DATA_BLOCK "Er"
TITLE =
VERSION : 0.1


  STRUCT
   KmA_DlmVF_GF { S7_m_c := 'true' }: BOOL ;	//GENERAL FAULT
   KmA_DlmVF_Strt { S7_m_c := 'true' }: BOOL ;	//FAULT START DELAY
   KmA_DlmVF_Stop { S7_m_c := 'true' }: BOOL ;	//FAULT STOP DELAY
   KmA_DlmVF_Trip { S7_m_c := 'true' }: BOOL ;	//FAULT TRIPPED
   KmA_Akt_GF { S7_m_c := 'true' }: BOOL ;	//GENERAL FAULT
   KmA_Akt_Strt { S7_m_c := 'true' }: BOOL ;	//FAULT START DELAY
   KmA_Akt_Stop { S7_m_c := 'true' }: BOOL ;	//FAULT STOP DELAY
   KmA_Akt_Trip { S7_m_c := 'true' }: BOOL ;	//FAULT TRIPPED
   KmA_SL_HL { S7_m_c := 'true' }: BOOL ;	//SILO HIGH LEVEL
   KmA_SL_LL { S7_m_c := 'true' }: BOOL ;	//SILO LOW LEVEL
   KmA_DlmKpk_GF { S7_m_c := 'true' }: BOOL ;	//GENERAL FAULT
   KmA_DlmKpk_Opn { S7_m_c := 'true' }: BOOL ;	//FAULT OPEN DELAY
   KmA_DlmKpk_Cls { S7_m_c := 'true' }: BOOL ;	//FAULT CLOSE DELAY
   KmA_DlmKpk_BthLmt { S7_m_c := 'true' }: BOOL ;	//BOTH LIMITS MADE
   KmA_BsltVF_GF { S7_m_c := 'true' }: BOOL ;	//GENERAL FAULT
   KmA_BsltVF_Strt { S7_m_c := 'true' }: BOOL ;	//FAULT START DELAY
   KmA_BsltVF_Stop { S7_m_c := 'true' }: BOOL ;	//FAULT STOP DELAY
   KmA_BsltVF_Trip { S7_m_c := 'true' }: BOOL ;	//FAULT TRIPPED
   KmA_BsltKpk_GF { S7_m_c := 'true' }: BOOL ;	//GENERAL FAULT
   KmA_BsltKpk_Opn { S7_m_c := 'true' }: BOOL ;	//FAULT OPEN DELAY
   KmA_BsltKpk_Cls { S7_m_c := 'true' }: BOOL ;	//FAULT CLOSE DELAY
   KmA_BsltKpk_BthLmt { S7_m_c := 'true' }: BOOL ;	//BOTH LIMITS MADE
   KmA_Ydk { S7_m_c := 'true' }: BOOL ;
   KmA_Ydk1 { S7_m_c := 'true' }: BOOL ;
   KmB_DlmVF_GF { S7_m_c := 'true' }: BOOL ;	//GENERAL FAULT
   KmB_DlmVF_Strt { S7_m_c := 'true' }: BOOL ;	//FAULT START DELAY
   KmB_DlmVF_Stop { S7_m_c := 'true' }: BOOL ;	//FAULT STOP DELAY
   KmB_DlmVF_Trip { S7_m_c := 'true' }: BOOL ;	//FAULT TRIPPED
   KmB_Akt_GF { S7_m_c := 'true' }: BOOL ;	//GENERAL FAULT
   KmB_Akt_Strt { S7_m_c := 'true' }: BOOL ;	//FAULT START DELAY
   KmB_Akt_Stop { S7_m_c := 'true' }: BOOL ;	//FAULT STOP DELAY
   KmB_Akt_Trip { S7_m_c := 'true' }: BOOL ;	//FAULT TRIPPED
   KmB_DlmKpk_GF { S7_m_c := 'true' }: BOOL ;	//GENERAL FAULT
   KmB_DlmKpk_Opn { S7_m_c := 'true' }: BOOL ;	//FAULT OPEN DELAY
   KmB_DlmKpk_Cls { S7_m_c := 'true' }: BOOL ;	//FAULT CLOSE DELAY
   KmB_DlmKpk_BthLmt { S7_m_c := 'true' }: BOOL ;	//BOTH LIMITS MADE
   KmB_SL_HL { S7_m_c := 'true' }: BOOL ;	//SILO HIGH LEVEL
   KmB_SL_LL { S7_m_c := 'true' }: BOOL ;	//SILO LOW LEVEL
   KmB_BsltVF_GF { S7_m_c := 'true' }: BOOL ;	//GENERAL FAULT
   KmB_BsltVF_Strt { S7_m_c := 'true' }: BOOL ;	//FAULT START DELAY
   KmB_BsltVF_Stop { S7_m_c := 'true' }: BOOL ;	//FAULT STOP DELAY
   KmB_BsltVF_Trip { S7_m_c := 'true' }: BOOL ;	//FAULT TRIPPED
   KmB_BsltKpk_GF { S7_m_c := 'true' }: BOOL ;	//GENERAL FAULT
   KmB_BsltKpk_Opn { S7_m_c := 'true' }: BOOL ;	//FAULT OPEN DELAY
   KmB_BsltKpk_Cls { S7_m_c := 'true' }: BOOL ;	//FAULT CLOSE DELAY
   KmB_BsltKpk_BthLmt { S7_m_c := 'true' }: BOOL ;	//BOTH LIMITS MADE
   KmB_Ydk { S7_m_c := 'true' }: BOOL ;
   KmB_Ydk1 { S7_m_c := 'true' }: BOOL ;
   SdA_DlmHlz_GF { S7_m_c := 'true' }: BOOL ;	//GENERAL FAULT
   SdA_DlmHlz_Strt { S7_m_c := 'true' }: BOOL ;	//FAULT START DELAY
   SdA_DlmHlz_Stop { S7_m_c := 'true' }: BOOL ;	//FAULT STOP DELAY
   SdA_DlmHlz_Trip { S7_m_c := 'true' }: BOOL ;	//FAULT TRIPPED
   SdA_Akt_GF { S7_m_c := 'true' }: BOOL ;	//GENERAL FAULT
   SdA_Akt_Strt { S7_m_c := 'true' }: BOOL ;	//FAULT START DELAY
   SdA_Akt_Stop { S7_m_c := 'true' }: BOOL ;	//FAULT STOP DELAY
   SdA_Akt_Trip { S7_m_c := 'true' }: BOOL ;	//FAULT TRIPPED
   SdA_SL_HL { S7_m_c := 'true' }: BOOL ;	//SILO HIGH LEVEL
   SdA_SL_LL { S7_m_c := 'true' }: BOOL ;	//SILO LOW LEVEL
   SdA_DlmKpk_GF { S7_m_c := 'true' }: BOOL ;	//GENERAL FAULT
   SdA_DlmKpk_Opn { S7_m_c := 'true' }: BOOL ;	//FAULT OPEN DELAY
   SdA_DlmKpk_Cls { S7_m_c := 'true' }: BOOL ;	//FAULT CLOSE DELAY
   SdA_DlmKpk_BthLmt { S7_m_c := 'true' }: BOOL ;	//BOTH LIMITS MADE
   SdB_DlmHlz_GF1 { S7_m_c := 'true' }: BOOL ;	//GENERAL FAULT
   SdB_DlmHlz_Strt { S7_m_c := 'true' }: BOOL ;	//FAULT START DELAY
   SdB_DlmHlz_Stop { S7_m_c := 'true' }: BOOL ;	//FAULT STOP DELAY
   SdB_DlmHlz_Trip { S7_m_c := 'true' }: BOOL ;	//FAULT TRIPPED
   SdB_Akt_GF { S7_m_c := 'true' }: BOOL ;	//GENERAL FAULT
   SdB_Akt_Strt { S7_m_c := 'true' }: BOOL ;	//FAULT START DELAY
   SdB_Akt_Stop { S7_m_c := 'true' }: BOOL ;	//FAULT STOP DELAY
   SdB_Akt_Trip { S7_m_c := 'true' }: BOOL ;	//FAULT TRIPPED
   SdB_SL_HL { S7_m_c := 'true' }: BOOL ;	//SILO HIGH LEVEL
   SdB_SL_LL { S7_m_c := 'true' }: BOOL ;	//SILO LOW LEVEL
   SdB_DlmKpk_GF { S7_m_c := 'true' }: BOOL ;	//GENERAL FAULT
   SdB_DlmKpk_Opn { S7_m_c := 'true' }: BOOL ;	//FAULT OPEN DELAY
   SdB_DlmKpk_Cls { S7_m_c := 'true' }: BOOL ;	//FAULT CLOSE DELAY
   SdB_DlmKpk_BthLmt { S7_m_c := 'true' }: BOOL ;	//BOTH LIMITS MADE
   Sd_BsltVF_GF { S7_m_c := 'true' }: BOOL ;	//GENERAL FAULT
   Sd_BsltVF_Strt { S7_m_c := 'true' }: BOOL ;	//FAULT START DELAY
   Sd_BsltVF_Stop { S7_m_c := 'true' }: BOOL ;	//FAULT STOP DELAY
   Sd_BsltVF_Trip { S7_m_c := 'true' }: BOOL ;	//FAULT TRIPPED
   Sd_BsltKpk_GF { S7_m_c := 'true' }: BOOL ;	//GENERAL FAULT
   Sd_BsltKpk_Opn { S7_m_c := 'true' }: BOOL ;	//FAULT OPEN DELAY
   Sd_BsltKpk_Cls { S7_m_c := 'true' }: BOOL ;	//FAULT CLOSE DELAY
   Sd_BsltKpk_BthLmt { S7_m_c := 'true' }: BOOL ;	//BOTH LIMITS MADE
   Sd_Ydk { S7_m_c := 'true' }: BOOL ;
   Sd_Ydk1 { S7_m_c := 'true' }: BOOL ;
   Sd_Ydk2 { S7_m_c := 'true' }: BOOL ;
   Sd_Ydk3 { S7_m_c := 'true' }: BOOL ;
   DlA_DlmHlz_GF { S7_m_c := 'true' }: BOOL ;	//GENERAL FAULT
   DlA_DlmHlz_Strt { S7_m_c := 'true' }: BOOL ;	//FAULT START DELAY
   DlA_DlmHlz_Stop { S7_m_c := 'true' }: BOOL ;	//FAULT STOP DELAY
   DlA_DlmHlz_Trip { S7_m_c := 'true' }: BOOL ;	//FAULT TRIPPED
   DlA_Akt_GF { S7_m_c := 'true' }: BOOL ;	//GENERAL FAULT
   DlA_Akt_Strt { S7_m_c := 'true' }: BOOL ;	//FAULT START DELAY
   DlA_Akt_Stop { S7_m_c := 'true' }: BOOL ;	//FAULT STOP DELAY
   DlA_Akt_Trip { S7_m_c := 'true' }: BOOL ;	//FAULT TRIPPED
   DlA_SL_HL { S7_m_c := 'true' }: BOOL ;	//SILO HIGH LEVEL
   DlA_SL_LL { S7_m_c := 'true' }: BOOL ;	//SILO LOW LEVEL
   DlA_DlmKpk_GF { S7_m_c := 'true' }: BOOL ;	//GENERAL FAULT
   DlA_DlmKpk_Opn { S7_m_c := 'true' }: BOOL ;	//FAULT OPEN DELAY
   DlA_DlmKpk_Cls { S7_m_c := 'true' }: BOOL ;	//FAULT CLOSE DELAY
   DlA_DlmKpk_BthLmt { S7_m_c := 'true' }: BOOL ;	//BOTH LIMITS MADE
   DlB_DlmHlz_GF { S7_m_c := 'true' }: BOOL ;	//GENERAL FAULT
   DlB_DlmHlz_Strt { S7_m_c := 'true' }: BOOL ;	//FAULT START DELAY
   DlB_DlmHlz_Stop { S7_m_c := 'true' }: BOOL ;	//FAULT STOP DELAY
   DlB_DlmHlz_Trip { S7_m_c := 'true' }: BOOL ;	//FAULT TRIPPED
   DlB_Akt_GF { S7_m_c := 'true' }: BOOL ;	//GENERAL FAULT
   DlB_Akt_Strt { S7_m_c := 'true' }: BOOL ;	//FAULT START DELAY
   DlB_Akt_Stop { S7_m_c := 'true' }: BOOL ;	//FAULT STOP DELAY
   DlB_Akt_Trip { S7_m_c := 'true' }: BOOL ;	//FAULT TRIPPED
   DlB_SL_HL { S7_m_c := 'true' }: BOOL ;	//SILO HIGH LEVEL
   DlB_SL_LL { S7_m_c := 'true' }: BOOL ;	//SILO LOW LEVEL
   DlB_DlmKpk_GF { S7_m_c := 'true' }: BOOL ;	//GENERAL FAULT
   DlB_DlmKpk_Opn { S7_m_c := 'true' }: BOOL ;	//FAULT OPEN DELAY
   DlB_DlmKpk_Cls { S7_m_c := 'true' }: BOOL ;	//FAULT CLOSE DELAY
   DlB_DlmKpk_BthLmt { S7_m_c := 'true' }: BOOL ;	//BOTH LIMITS MADE
   Dl_BsltHlz1_GF { S7_m_c := 'true' }: BOOL ;	//GENERAL FAULT
   Dl_BsltHlz1_Strt { S7_m_c := 'true' }: BOOL ;	//FAULT START DELAY
   Dl_BsltHlz1_Stop { S7_m_c := 'true' }: BOOL ;	//FAULT STOP DELAY
   Dl_BsltHlz1_Trip { S7_m_c := 'true' }: BOOL ;	//FAULT TRIPPED
   Dl_BsltHlz2_GF { S7_m_c := 'true' }: BOOL ;	//GENERAL FAULT
   Dl_BsltHlz2_Strt { S7_m_c := 'true' }: BOOL ;	//FAULT START DELAY
   Dl_BsltHlz2_Stop { S7_m_c := 'true' }: BOOL ;	//FAULT STOP DELAY
   Dl_BsltHlz2_Trip { S7_m_c := 'true' }: BOOL ;	//FAULT TRIPPED
   Dl_BsltKpk_GF { S7_m_c := 'true' }: BOOL ;	//GENERAL FAULT
   Dl_BsltKpk_Opn { S7_m_c := 'true' }: BOOL ;	//FAULT OPEN DELAY
   Dl_BsltKpk_Cls { S7_m_c := 'true' }: BOOL ;	//FAULT CLOSE DELAY
   Dl_BsltKpk_BthLmt { S7_m_c := 'true' }: BOOL ;	//BOTH LIMITS MADE
   Kl_DlmHlz_GF { S7_m_c := 'true' }: BOOL ;	//GENERAL FAULT
   Kl_DlmHlz_Strt { S7_m_c := 'true' }: BOOL ;	//FAULT START DELAY
   Kl_DlmHlz_Stop { S7_m_c := 'true' }: BOOL ;	//FAULT STOP DELAY
   Kl_DlmHlz_Trip { S7_m_c := 'true' }: BOOL ;	//FAULT TRIPPED
   Kl_Akt_GF { S7_m_c := 'true' }: BOOL ;	//GENERAL FAULT
   Kl_Akt_Strt { S7_m_c := 'true' }: BOOL ;	//FAULT START DELAY
   Kl_Akt_Stop { S7_m_c := 'true' }: BOOL ;	//FAULT STOP DELAY
   Kl_Akt_Trip { S7_m_c := 'true' }: BOOL ;	//FAULT TRIPPED
   Kl_SL_HL { S7_m_c := 'true' }: BOOL ;	//SILO HIGH LEVEL
   Kl_SL_LL { S7_m_c := 'true' }: BOOL ;	//SILO LOW LEVEL
   Kl_DlmKpk_GF { S7_m_c := 'true' }: BOOL ;	//GENERAL FAULT
   Kl_DlmKpk_Opn { S7_m_c := 'true' }: BOOL ;	//FAULT OPEN DELAY
   Kl_DlmKpk_Cls { S7_m_c := 'true' }: BOOL ;	//FAULT CLOSE DELAY
   Kl_DlmKpk_BthLmt { S7_m_c := 'true' }: BOOL ;	//BOTH LIMITS MADE
   Kl_BsltVF_GF { S7_m_c := 'true' }: BOOL ;	//GENERAL FAULT
   Kl_BsltVF_Strt { S7_m_c := 'true' }: BOOL ;	//FAULT START DELAY
   Kl_BsltVF_Stop { S7_m_c := 'true' }: BOOL ;	//FAULT STOP DELAY
   Kl_BsltVF_Trip { S7_m_c := 'true' }: BOOL ;	//FAULT TRIPPED
   Kl_BsltKpk_GF { S7_m_c := 'true' }: BOOL ;	//GENERAL FAULT
   Kl_BsltKpk_Opn { S7_m_c := 'true' }: BOOL ;	//FAULT OPEN DELAY
   Kl_BsltKpk_Cls { S7_m_c := 'true' }: BOOL ;	//FAULT CLOSE DELAY
   Kl_BsltKpk_BthLmt { S7_m_c := 'true' }: BOOL ;	//BOTH LIMITS MADE
   Kl_Ydk { S7_m_c := 'true' }: BOOL ;
   Kl_Ydk1 { S7_m_c := 'true' }: BOOL ;
   FlA_DlmHlz_GF { S7_m_c := 'true' }: BOOL ;	//GENERAL FAULT
   FlA_DlmHlz_Strt { S7_m_c := 'true' }: BOOL ;	//FAULT START DELAY
   FlA_DlmHlz_Stop { S7_m_c := 'true' }: BOOL ;	//FAULT STOP DELAY
   FlA_DlmHlz_Trip { S7_m_c := 'true' }: BOOL ;	//FAULT TRIPPED
   FlA_Akt_GF { S7_m_c := 'true' }: BOOL ;	//GENERAL FAULT
   FlA_Akt_Strt { S7_m_c := 'true' }: BOOL ;	//FAULT START DELAY
   FlA_Akt_Stop { S7_m_c := 'true' }: BOOL ;	//FAULT STOP DELAY
   FlA_Akt_Trip { S7_m_c := 'true' }: BOOL ;	//FAULT TRIPPED
   FlA_SL_HL { S7_m_c := 'true' }: BOOL ;	//SILO HIGH LEVEL
   FlA_SL_LL { S7_m_c := 'true' }: BOOL ;	//SILO LOW LEVEL
   FlA_DlmKpk_GF { S7_m_c := 'true' }: BOOL ;	//GENERAL FAULT
   FlA_DlmKpk_Opn { S7_m_c := 'true' }: BOOL ;	//FAULT OPEN DELAY
   FlA_DlmKpk_Cls { S7_m_c := 'true' }: BOOL ;	//FAULT CLOSE DELAY
   FlA_DlmKpk_BthLmt { S7_m_c := 'true' }: BOOL ;	//BOTH LIMITS MADE
   FlB_DlmHlz_GF { S7_m_c := 'true' }: BOOL ;	//GENERAL FAULT
   FlB_DlmHlz_Strt { S7_m_c := 'true' }: BOOL ;	//FAULT START DELAY
   FlB_DlmHlz_Stop { S7_m_c := 'true' }: BOOL ;	//FAULT STOP DELAY
   FlB_DlmHlz_Trip { S7_m_c := 'true' }: BOOL ;	//FAULT TRIPPED
   FlB_Akt_GF { S7_m_c := 'true' }: BOOL ;	//GENERAL FAULT
   FlB_Akt_Strt { S7_m_c := 'true' }: BOOL ;	//FAULT START DELAY
   FlB_Akt_Stop { S7_m_c := 'true' }: BOOL ;	//FAULT STOP DELAY
   FlB_Akt_Trip { S7_m_c := 'true' }: BOOL ;	//FAULT TRIPPED
   FlB_SL_HL { S7_m_c := 'true' }: BOOL ;	//SILO HIGH LEVEL
   FlB_SL_LL { S7_m_c := 'true' }: BOOL ;	//SILO LOW LEVEL
   FlB_DlmKpk_GF { S7_m_c := 'true' }: BOOL ;	//GENERAL FAULT
   FlB_DlmKpk_Opn { S7_m_c := 'true' }: BOOL ;	//FAULT OPEN DELAY
   FlB_DlmKpk_Cls { S7_m_c := 'true' }: BOOL ;	//FAULT CLOSE DELAY
   FlB_DlmKpk_BthLmt { S7_m_c := 'true' }: BOOL ;	//BOTH LIMITS MADE
   Fl_BsltVF_GF { S7_m_c := 'true' }: BOOL ;	//GENERAL FAULT
   Fl_BsltVF_Strt { S7_m_c := 'true' }: BOOL ;	//FAULT START DELAY
   Fl_BsltVF_Stop { S7_m_c := 'true' }: BOOL ;	//FAULT STOP DELAY
   Fl_BsltVF_Trip { S7_m_c := 'true' }: BOOL ;	//FAULT TRIPPED
   Fl_BsltKpk_GF { S7_m_c := 'true' }: BOOL ;	//GENERAL FAULT
   Fl_BsltKpk_Opn { S7_m_c := 'true' }: BOOL ;	//FAULT OPEN DELAY
   Fl_BsltKpk_Cls { S7_m_c := 'true' }: BOOL ;	//FAULT CLOSE DELAY
   Fl_BsltKpk_BthLmt { S7_m_c := 'true' }: BOOL ;	//BOTH LIMITS MADE
   Fl_Ydk { S7_m_c := 'true' }: BOOL ;
   Fl_Ydk1 { S7_m_c := 'true' }: BOOL ;
   Fl_Ydk2 { S7_m_c := 'true' }: BOOL ;
   Fl_Ydk3 { S7_m_c := 'true' }: BOOL ;
   Sl_DlmHlz_GF { S7_m_c := 'true' }: BOOL ;	//GENERAL FAULT
   Sl_DlmHlz_Strt { S7_m_c := 'true' }: BOOL ;	//FAULT START DELAY
   Sl_DlmHlz_Stop { S7_m_c := 'true' }: BOOL ;	//FAULT STOP DELAY
   Sl_DlmHlz_Trip { S7_m_c := 'true' }: BOOL ;	//FAULT TRIPPED
   Sl_Akt_GF { S7_m_c := 'true' }: BOOL ;	//GENERAL FAULT
   Sl_Akt_Strt { S7_m_c := 'true' }: BOOL ;	//FAULT START DELAY
   Sl_Akt_Stop { S7_m_c := 'true' }: BOOL ;	//FAULT STOP DELAY
   Sl_Akt_Trip { S7_m_c := 'true' }: BOOL ;	//FAULT TRIPPED
   Sl_SL_HL { S7_m_c := 'true' }: BOOL ;	//SILO HIGH LEVEL
   Sl_SL_LL { S7_m_c := 'true' }: BOOL ;	//SILO LOW LEVEL
   Sl_DlmKpk_GF { S7_m_c := 'true' }: BOOL ;	//GENERAL FAULT
   Sl_DlmKpk_Opn { S7_m_c := 'true' }: BOOL ;	//FAULT OPEN DELAY
   Sl_DlmKpk_Cls { S7_m_c := 'true' }: BOOL ;	//FAULT CLOSE DELAY
   Sl_DlmKpk_BthLmt { S7_m_c := 'true' }: BOOL ;	//BOTH LIMITS MADE
   Sl_BsltVF_GF { S7_m_c := 'true' }: BOOL ;	//GENERAL FAULT
   Sl_BsltVF_Strt { S7_m_c := 'true' }: BOOL ;	//FAULT START DELAY
   Sl_BsltVF_Stop { S7_m_c := 'true' }: BOOL ;	//FAULT STOP DELAY
   Sl_BsltVF_Trip { S7_m_c := 'true' }: BOOL ;	//FAULT TRIPPED
   Sl_BsltKpk_GF { S7_m_c := 'true' }: BOOL ;	//GENERAL FAULT
   Sl_BsltKpk_Opn { S7_m_c := 'true' }: BOOL ;	//FAULT OPEN DELAY
   Sl_BsltKpk_Cls { S7_m_c := 'true' }: BOOL ;	//FAULT CLOSE DELAY
   Sl_BsltKpk_BthLmt { S7_m_c := 'true' }: BOOL ;	//BOTH LIMITS MADE
   Sl_Ydk { S7_m_c := 'true' }: BOOL ;
   Sl_Ydk1 { S7_m_c := 'true' }: BOOL ;
   Hm_DlmHlz_GF { S7_m_c := 'true' }: BOOL ;	//GENERAL FAULT
   Hm_DlmHlz_Strt { S7_m_c := 'true' }: BOOL ;	//FAULT START DELAY
   Hm_DlmHlz_Stop { S7_m_c := 'true' }: BOOL ;	//FAULT STOP DELAY
   Hm_DlmHlz_Trip { S7_m_c := 'true' }: BOOL ;	//FAULT TRIPPED
   Hm_Akt_GF { S7_m_c := 'true' }: BOOL ;	//GENERAL FAULT
   Hm_Akt_Strt { S7_m_c := 'true' }: BOOL ;	//FAULT START DELAY
   Hm_Akt_Stop { S7_m_c := 'true' }: BOOL ;	//FAULT STOP DELAY
   Hm_Akt_Trip { S7_m_c := 'true' }: BOOL ;	//FAULT TRIPPED
   Hm_SL_HL { S7_m_c := 'true' }: BOOL ;	//SILO HIGH LEVEL
   Hm_SL_LL { S7_m_c := 'true' }: BOOL ;	//SILO LOW LEVEL
   Hm_DlmKpk_GF { S7_m_c := 'true' }: BOOL ;	//GENERAL FAULT
   Hm_DlmKpk_Opn { S7_m_c := 'true' }: BOOL ;	//FAULT OPEN DELAY
   Hm_DlmKpk_Cls { S7_m_c := 'true' }: BOOL ;	//FAULT CLOSE DELAY
   Hm_DlmKpk_BthLmt { S7_m_c := 'true' }: BOOL ;	//BOTH LIMITS MADE
   Hm_BsltVF_GF { S7_m_c := 'true' }: BOOL ;	//GENERAL FAULT
   Hm_BsltVF_Strt { S7_m_c := 'true' }: BOOL ;	//FAULT START DELAY
   Hm_BsltVF_Stop { S7_m_c := 'true' }: BOOL ;	//FAULT STOP DELAY
   Hm_BsltVF_Trip { S7_m_c := 'true' }: BOOL ;	//FAULT TRIPPED
   Hm_BsltKpk_GF { S7_m_c := 'true' }: BOOL ;	//GENERAL FAULT
   Hm_BsltKpk_Opn { S7_m_c := 'true' }: BOOL ;	//FAULT OPEN DELAY
   Hm_BsltKpk_Cls { S7_m_c := 'true' }: BOOL ;	//FAULT CLOSE DELAY
   Hm_BsltKpk_BthLmt { S7_m_c := 'true' }: BOOL ;	//BOTH LIMITS MADE
   Hm_Ydk { S7_m_c := 'true' }: BOOL ;
   Hm_Ydk1 { S7_m_c := 'true' }: BOOL ;
   An_DlmHlz_GF { S7_m_c := 'true' }: BOOL ;	//GENERAL FAULT
   An_DlmHlz_Strt { S7_m_c := 'true' }: BOOL ;	//FAULT START DELAY
   An_DlmHlz_Stop { S7_m_c := 'true' }: BOOL ;	//FAULT STOP DELAY
   An_DlmHlz_Trip { S7_m_c := 'true' }: BOOL ;	//FAULT TRIPPED
   An_Akt_GF { S7_m_c := 'true' }: BOOL ;	//GENERAL FAULT
   An_Akt_Strt { S7_m_c := 'true' }: BOOL ;	//FAULT START DELAY
   An_Akt_Stop { S7_m_c := 'true' }: BOOL ;	//FAULT STOP DELAY
   An_Akt_Trip { S7_m_c := 'true' }: BOOL ;	//FAULT TRIPPED
   An_SL_HL { S7_m_c := 'true' }: BOOL ;	//SILO HIGH LEVEL
   An_SL_LL { S7_m_c := 'true' }: BOOL ;	//SILO LOW LEVEL
   An_DlmKpk_GF { S7_m_c := 'true' }: BOOL ;	//GENERAL FAULT
   An_DlmKpk_Opn { S7_m_c := 'true' }: BOOL ;	//FAULT OPEN DELAY
   An_DlmKpk_Cls { S7_m_c := 'true' }: BOOL ;	//FAULT CLOSE DELAY
   An_DlmKpk_BthLmt { S7_m_c := 'true' }: BOOL ;	//BOTH LIMITS MADE
   An_BsltKrs_GF { S7_m_c := 'true' }: BOOL ;	//GENERAL FAULT
   An_BsltKrs_Strt { S7_m_c := 'true' }: BOOL ;	//FAULT START DELAY
   An_BsltKrs_Stop { S7_m_c := 'true' }: BOOL ;	//FAULT STOP DELAY
   An_BsltKrs_Trip { S7_m_c := 'true' }: BOOL ;	//FAULT TRIPPED
   An_BsltHlz_GF { S7_m_c := 'true' }: BOOL ;	//GENERAL FAULT
   An_BsltHlz_Strt { S7_m_c := 'true' }: BOOL ;	//FAULT START DELAY
   An_BsltHlz_Stop { S7_m_c := 'true' }: BOOL ;	//FAULT STOP DELAY
   An_BsltHlz_Trip { S7_m_c := 'true' }: BOOL ;	//FAULT TRIPPED
   An_BsltKpk_GF { S7_m_c := 'true' }: BOOL ;	//GENERAL FAULT
   An_BsltKpk_Opn { S7_m_c := 'true' }: BOOL ;	//FAULT OPEN DELAY
   An_BsltKpk_Cls { S7_m_c := 'true' }: BOOL ;	//FAULT CLOSE DELAY
   An_BsltKpk_BthLmt { S7_m_c := 'true' }: BOOL ;	//BOTH LIMITS MADE
   An_Ydk { S7_m_c := 'true' }: BOOL ;
   An_Ydk1 { S7_m_c := 'true' }: BOOL ;
   An_Ydk2 { S7_m_c := 'true' }: BOOL ;
   An_Ydk3 { S7_m_c := 'true' }: BOOL ;
   An_Ydk4 { S7_m_c := 'true' }: BOOL ;
   An_Ydk5 { S7_m_c := 'true' }: BOOL ;
   e83_TopBnd_GF { S7_m_c := 'true' }: BOOL ;	//GENERAL FAULT
   e83_TopBnd_Strt { S7_m_c := 'true' }: BOOL ;	//FAULT START DELAY
   e83_TopBnd_Stop { S7_m_c := 'true' }: BOOL ;	//FAULT STOP DELAY
   e83_TopBnd_Trip { S7_m_c := 'true' }: BOOL ;	//FAULT TRIPPED
   e83_LmtSwtch { S7_m_c := 'true' }: BOOL ;	//CONVEYOR BAND LIMIT SWITCH ERROR
   e83_EmrSwtch { S7_m_c := 'true' }: BOOL ;	//CONVEYOR BAND EMERGENCY SWITCH ERROR
   e83_MovingSnsr { S7_m_c := 'true' }: BOOL ;	//CONVEYOR BAND MOVING SENSOR ERROR
   e83_Ydk { S7_m_c := 'true' }: BOOL ;	//CONVEYOR BAND MOVING SENSOR ERROR
   e83_Fan_GF { S7_m_c := 'true' }: BOOL ;	//GENERAL FAULT
   e83_Fan_Strt { S7_m_c := 'true' }: BOOL ;	//FAULT START DELAY
   e83_Fan_Stop { S7_m_c := 'true' }: BOOL ;	//FAULT STOP DELAY
   e83_Fan_Trip { S7_m_c := 'true' }: BOOL ;	//FAULT TRIPPED
   e83_Ydk1 { S7_m_c := 'true' }: BOOL ;	//CONVEYOR BAND MOVING SENSOR ERROR
   e83_Ydk2 { S7_m_c := 'true' }: BOOL ;	//CONVEYOR BAND MOVING SENSOR ERROR
   e83_Ydk3 { S7_m_c := 'true' }: BOOL ;	//CONVEYOR BAND MOVING SENSOR ERROR
   e83_Ydk4 { S7_m_c := 'true' }: BOOL ;	//CONVEYOR BAND MOVING SENSOR ERROR
   e87_Bnd_GF { S7_m_c := 'true' }: BOOL ;	//GENERAL FAULT
   e87_Bnd_Strt { S7_m_c := 'true' }: BOOL ;	//FAULT START DELAY
   e87_Bnd_Stop { S7_m_c := 'true' }: BOOL ;	//FAULT STOP DELAY
   e87_Bnd_Trip { S7_m_c := 'true' }: BOOL ;	//FAULT TRIPPED
   e87_LmtSwtch { S7_m_c := 'true' }: BOOL ;	//CONVEYOR BAND LIMIT SWITCH ERROR
   e87_EmrSwtch { S7_m_c := 'true' }: BOOL ;	//CONVEYOR BAND EMERGENCY SWITCH ERROR
   e87_MovingSnsr { S7_m_c := 'true' }: BOOL ;	//CONVEYOR BAND MOVING SENSOR ERROR
   e87_Ydk { S7_m_c := 'true' }: BOOL ;	//CONVEYOR BAND MOVING SENSOR ERROR
   e87_Fan_GF { S7_m_c := 'true' }: BOOL ;	//GENERAL FAULT
   e87_Fan_Strt { S7_m_c := 'true' }: BOOL ;	//FAULT START DELAY
   e87_Fan_Stop { S7_m_c := 'true' }: BOOL ;	//FAULT STOP DELAY
   e87_Fan_Trip { S7_m_c := 'true' }: BOOL ;	//FAULT TRIPPED
   e87_Ydk1 { S7_m_c := 'true' }: BOOL ;	//CONVEYOR BAND MOVING SENSOR ERROR
   e87_Ydk2 { S7_m_c := 'true' }: BOOL ;	//CONVEYOR BAND MOVING SENSOR ERROR
   e87_Ydk3 { S7_m_c := 'true' }: BOOL ;	//CONVEYOR BAND MOVING SENSOR ERROR
   e87_Ydk4 { S7_m_c := 'true' }: BOOL ;	//CONVEYOR BAND MOVING SENSOR ERROR
   TozTopFan_GF1 { S7_m_c := 'true' }: BOOL ;	//GENERAL FAULT
   TozTopFan_Strt1 { S7_m_c := 'true' }: BOOL ;	//FAULT START DELAY
   TozTopFan_Stop1 { S7_m_c := 'true' }: BOOL ;	//FAULT STOP DELAY
   TozTopFan_Trip1 { S7_m_c := 'true' }: BOOL ;	//FAULT TRIPPED
   Ydk { S7_m_c := 'true' }: BOOL ;	//FAULT TRIPPED
   Ydk1 { S7_m_c := 'true' }: BOOL ;	//FAULT TRIPPED
   Ydk2 { S7_m_c := 'true' }: BOOL ;	//FAULT TRIPPED
   Ydk3 { S7_m_c := 'true' }: BOOL ;	//FAULT TRIPPED
   TolErrKmADlm { S7_m_c := 'true' }: BOOL ;	//TOLERANS ERROR FILLING
   TolErrKmABslt { S7_m_c := 'true' }: BOOL ;	//TOLERANS ERROR DISCHARGE
   TolErrKmBDlm { S7_m_c := 'true' }: BOOL ;	//TOLERANS ERROR FILLING
   TolErrKmBBslt { S7_m_c := 'true' }: BOOL ;	//TOLERANS ERROR DISCHARGE
   TolErrSdADlm { S7_m_c := 'true' }: BOOL ;	//TOLERANS ERROR FILLING
   TolErrSdBDlm { S7_m_c := 'true' }: BOOL ;	//TOLERANS ERROR FILLING
   TolErrSdBslt { S7_m_c := 'true' }: BOOL ;	//TOLERANS ERROR DISCHARGE
   TolErrDlADlm { S7_m_c := 'true' }: BOOL ;	//TOLERANS ERROR FILLING
   TolErrDlBDlm { S7_m_c := 'true' }: BOOL ;	//TOLERANS ERROR FILLING
   TolErrDlBslt { S7_m_c := 'true' }: BOOL ;	//TOLERANS ERROR DISCHARGE
   TolErrKlDlm { S7_m_c := 'true' }: BOOL ;	//TOLERANS ERROR FILLING
   TolErrKlBslt { S7_m_c := 'true' }: BOOL ;	//TOLERANS ERROR DISCHARGE
   TolErrFlADlm { S7_m_c := 'true' }: BOOL ;	//TOLERANS ERROR FILLING
   TolErrFlBDlm { S7_m_c := 'true' }: BOOL ;	//TOLERANS ERROR FILLING
   TolErrFlBslt { S7_m_c := 'true' }: BOOL ;	//TOLERANS ERROR DISCHARGE
   TolErrSlDlm { S7_m_c := 'true' }: BOOL ;	//TOLERANS ERROR FILLING
   TolErrSlBslt { S7_m_c := 'true' }: BOOL ;	//TOLERANS ERROR DISCHARGE
   TolErrHmDlm { S7_m_c := 'true' }: BOOL ;	//TOLERANS ERROR FILLING
   TolErrHmBslt { S7_m_c := 'true' }: BOOL ;	//TOLERANS ERROR DISCHARGE
   TolErrAnDlm { S7_m_c := 'true' }: BOOL ;	//TOLERANS ERROR FILLING
   TolErrAnBslt { S7_m_c := 'true' }: BOOL ;	//TOLERANS ERROR DISCHARGE
   TolErrTopKntr { S7_m_c := 'true' }: BOOL ;	//TOLERANS ERROR
   TolErrYdk { S7_m_c := 'true' }: BOOL ;	//TOLERANS ERROR
   TolErrYdk1 { S7_m_c := 'true' }: BOOL ;	//TOLERANS ERROR
   BX3_ErrKmA { S7_m_c := 'true' }: BOOL ;	//BX3 ERROR
   BX3_ErrKmB { S7_m_c := 'true' }: BOOL ;	//BX3 ERROR
   BX3_ErrSd { S7_m_c := 'true' }: BOOL ;	//BX3 ERROR
   BX3_ErrDl { S7_m_c := 'true' }: BOOL ;	//BX3 ERROR
   BX3_ErrKl { S7_m_c := 'true' }: BOOL ;	//BX3 ERROR
   BX3_ErrFl { S7_m_c := 'true' }: BOOL ;	//BX3 ERROR
   BX3_ErrSl { S7_m_c := 'true' }: BOOL ;	//BX3 ERROR
   BX3_ErrHm { S7_m_c := 'true' }: BOOL ;	//BX3 ERROR
   BX3_ErrAn { S7_m_c := 'true' }: BOOL ;	//BX3 ERROR
   BX3_ErrYdk { S7_m_c := 'true' }: BOOL ;	//BX3 ERROR
   BX3_ErrYdk1 { S7_m_c := 'true' }: BOOL ;	//BX3 ERROR
   BX3_ErrYdk2 { S7_m_c := 'true' }: BOOL ;	//BX3 ERROR
   BX3_ErrYdk3 { S7_m_c := 'true' }: BOOL ;	//BX3 ERROR
   BX3_ErrYdk4 { S7_m_c := 'true' }: BOOL ;	//BX3 ERROR
   BX3_ErrYdk5 { S7_m_c := 'true' }: BOOL ;	//BX3 ERROR
   BX3_ErrYdk6 { S7_m_c := 'true' }: BOOL ;	//BX3 ERROR
  END_STRUCT ;
BEGIN
   KmA_DlmVF_GF := FALSE;
   KmA_DlmVF_Strt := FALSE;
   KmA_DlmVF_Stop := FALSE;
   KmA_DlmVF_Trip := FALSE;
   KmA_Akt_GF := FALSE;
   KmA_Akt_Strt := FALSE;
   KmA_Akt_Stop := FALSE;
   KmA_Akt_Trip := FALSE;
   KmA_SL_HL := FALSE;
   KmA_SL_LL := FALSE;
   KmA_DlmKpk_GF := FALSE;
   KmA_DlmKpk_Opn := FALSE;
   KmA_DlmKpk_Cls := FALSE;
   KmA_DlmKpk_BthLmt := FALSE;
   KmA_BsltVF_GF := FALSE;
   KmA_BsltVF_Strt := FALSE;
   KmA_BsltVF_Stop := FALSE;
   KmA_BsltVF_Trip := FALSE;
   KmA_BsltKpk_GF := FALSE;
   KmA_BsltKpk_Opn := FALSE;
   KmA_BsltKpk_Cls := FALSE;
   KmA_BsltKpk_BthLmt := FALSE;
   KmA_Ydk := FALSE;
   KmA_Ydk1 := FALSE;
   KmB_DlmVF_GF := FALSE;
   KmB_DlmVF_Strt := FALSE;
   KmB_DlmVF_Stop := FALSE;
   KmB_DlmVF_Trip := FALSE;
   KmB_Akt_GF := FALSE;
   KmB_Akt_Strt := FALSE;
   KmB_Akt_Stop := FALSE;
   KmB_Akt_Trip := FALSE;
   KmB_DlmKpk_GF := FALSE;
   KmB_DlmKpk_Opn := FALSE;
   KmB_DlmKpk_Cls := FALSE;
   KmB_DlmKpk_BthLmt := FALSE;
   KmB_SL_HL := FALSE;
   KmB_SL_LL := FALSE;
   KmB_BsltVF_GF := FALSE;
   KmB_BsltVF_Strt := FALSE;
   KmB_BsltVF_Stop := FALSE;
   KmB_BsltVF_Trip := FALSE;
   KmB_BsltKpk_GF := FALSE;
   KmB_BsltKpk_Opn := FALSE;
   KmB_BsltKpk_Cls := FALSE;
   KmB_BsltKpk_BthLmt := FALSE;
   KmB_Ydk := FALSE;
   KmB_Ydk1 := FALSE;
   SdA_DlmHlz_GF := FALSE;
   SdA_DlmHlz_Strt := FALSE;
   SdA_DlmHlz_Stop := FALSE;
   SdA_DlmHlz_Trip := FALSE;
   SdA_Akt_GF := FALSE;
   SdA_Akt_Strt := FALSE;
   SdA_Akt_Stop := FALSE;
   SdA_Akt_Trip := FALSE;
   SdA_SL_HL := FALSE;
   SdA_SL_LL := FALSE;
   SdA_DlmKpk_GF := FALSE;
   SdA_DlmKpk_Opn := FALSE;
   SdA_DlmKpk_Cls := FALSE;
   SdA_DlmKpk_BthLmt := FALSE;
   SdB_DlmHlz_GF1 := FALSE;
   SdB_DlmHlz_Strt := FALSE;
   SdB_DlmHlz_Stop := FALSE;
   SdB_DlmHlz_Trip := FALSE;
   SdB_Akt_GF := FALSE;
   SdB_Akt_Strt := FALSE;
   SdB_Akt_Stop := FALSE;
   SdB_Akt_Trip := FALSE;
   SdB_SL_HL := FALSE;
   SdB_SL_LL := FALSE;
   SdB_DlmKpk_GF := FALSE;
   SdB_DlmKpk_Opn := FALSE;
   SdB_DlmKpk_Cls := FALSE;
   SdB_DlmKpk_BthLmt := FALSE;
   Sd_BsltVF_GF := FALSE;
   Sd_BsltVF_Strt := FALSE;
   Sd_BsltVF_Stop := FALSE;
   Sd_BsltVF_Trip := FALSE;
   Sd_BsltKpk_GF := FALSE;
   Sd_BsltKpk_Opn := FALSE;
   Sd_BsltKpk_Cls := FALSE;
   Sd_BsltKpk_BthLmt := FALSE;
   Sd_Ydk := FALSE;
   Sd_Ydk1 := FALSE;
   Sd_Ydk2 := FALSE;
   Sd_Ydk3 := FALSE;
   DlA_DlmHlz_GF := FALSE;
   DlA_DlmHlz_Strt := FALSE;
   DlA_DlmHlz_Stop := FALSE;
   DlA_DlmHlz_Trip := FALSE;
   DlA_Akt_GF := FALSE;
   DlA_Akt_Strt := FALSE;
   DlA_Akt_Stop := FALSE;
   DlA_Akt_Trip := FALSE;
   DlA_SL_HL := FALSE;
   DlA_SL_LL := FALSE;
   DlA_DlmKpk_GF := FALSE;
   DlA_DlmKpk_Opn := FALSE;
   DlA_DlmKpk_Cls := FALSE;
   DlA_DlmKpk_BthLmt := FALSE;
   DlB_DlmHlz_GF := FALSE;
   DlB_DlmHlz_Strt := FALSE;
   DlB_DlmHlz_Stop := FALSE;
   DlB_DlmHlz_Trip := FALSE;
   DlB_Akt_GF := FALSE;
   DlB_Akt_Strt := FALSE;
   DlB_Akt_Stop := FALSE;
   DlB_Akt_Trip := FALSE;
   DlB_SL_HL := FALSE;
   DlB_SL_LL := FALSE;
   DlB_DlmKpk_GF := FALSE;
   DlB_DlmKpk_Opn := FALSE;
   DlB_DlmKpk_Cls := FALSE;
   DlB_DlmKpk_BthLmt := FALSE;
   Dl_BsltHlz1_GF := FALSE;
   Dl_BsltHlz1_Strt := FALSE;
   Dl_BsltHlz1_Stop := FALSE;
   Dl_BsltHlz1_Trip := FALSE;
   Dl_BsltHlz2_GF := FALSE;
   Dl_BsltHlz2_Strt := FALSE;
   Dl_BsltHlz2_Stop := FALSE;
   Dl_BsltHlz2_Trip := FALSE;
   Dl_BsltKpk_GF := FALSE;
   Dl_BsltKpk_Opn := FALSE;
   Dl_BsltKpk_Cls := FALSE;
   Dl_BsltKpk_BthLmt := FALSE;
   Kl_DlmHlz_GF := FALSE;
   Kl_DlmHlz_Strt := FALSE;
   Kl_DlmHlz_Stop := FALSE;
   Kl_DlmHlz_Trip := FALSE;
   Kl_Akt_GF := FALSE;
   Kl_Akt_Strt := FALSE;
   Kl_Akt_Stop := FALSE;
   Kl_Akt_Trip := FALSE;
   Kl_SL_HL := FALSE;
   Kl_SL_LL := FALSE;
   Kl_DlmKpk_GF := FALSE;
   Kl_DlmKpk_Opn := FALSE;
   Kl_DlmKpk_Cls := FALSE;
   Kl_DlmKpk_BthLmt := FALSE;
   Kl_BsltVF_GF := FALSE;
   Kl_BsltVF_Strt := FALSE;
   Kl_BsltVF_Stop := FALSE;
   Kl_BsltVF_Trip := FALSE;
   Kl_BsltKpk_GF := FALSE;
   Kl_BsltKpk_Opn := FALSE;
   Kl_BsltKpk_Cls := FALSE;
   Kl_BsltKpk_BthLmt := FALSE;
   Kl_Ydk := FALSE;
   Kl_Ydk1 := FALSE;
   FlA_DlmHlz_GF := FALSE;
   FlA_DlmHlz_Strt := FALSE;
   FlA_DlmHlz_Stop := FALSE;
   FlA_DlmHlz_Trip := FALSE;
   FlA_Akt_GF := FALSE;
   FlA_Akt_Strt := FALSE;
   FlA_Akt_Stop := FALSE;
   FlA_Akt_Trip := FALSE;
   FlA_SL_HL := FALSE;
   FlA_SL_LL := FALSE;
   FlA_DlmKpk_GF := FALSE;
   FlA_DlmKpk_Opn := FALSE;
   FlA_DlmKpk_Cls := FALSE;
   FlA_DlmKpk_BthLmt := FALSE;
   FlB_DlmHlz_GF := FALSE;
   FlB_DlmHlz_Strt := FALSE;
   FlB_DlmHlz_Stop := FALSE;
   FlB_DlmHlz_Trip := FALSE;
   FlB_Akt_GF := FALSE;
   FlB_Akt_Strt := FALSE;
   FlB_Akt_Stop := FALSE;
   FlB_Akt_Trip := FALSE;
   FlB_SL_HL := FALSE;
   FlB_SL_LL := FALSE;
   FlB_DlmKpk_GF := FALSE;
   FlB_DlmKpk_Opn := FALSE;
   FlB_DlmKpk_Cls := FALSE;
   FlB_DlmKpk_BthLmt := FALSE;
   Fl_BsltVF_GF := FALSE;
   Fl_BsltVF_Strt := FALSE;
   Fl_BsltVF_Stop := FALSE;
   Fl_BsltVF_Trip := FALSE;
   Fl_BsltKpk_GF := FALSE;
   Fl_BsltKpk_Opn := FALSE;
   Fl_BsltKpk_Cls := FALSE;
   Fl_BsltKpk_BthLmt := FALSE;
   Fl_Ydk := FALSE;
   Fl_Ydk1 := FALSE;
   Fl_Ydk2 := FALSE;
   Fl_Ydk3 := FALSE;
   Sl_DlmHlz_GF := FALSE;
   Sl_DlmHlz_Strt := FALSE;
   Sl_DlmHlz_Stop := FALSE;
   Sl_DlmHlz_Trip := FALSE;
   Sl_Akt_GF := FALSE;
   Sl_Akt_Strt := FALSE;
   Sl_Akt_Stop := FALSE;
   Sl_Akt_Trip := FALSE;
   Sl_SL_HL := FALSE;
   Sl_SL_LL := FALSE;
   Sl_DlmKpk_GF := FALSE;
   Sl_DlmKpk_Opn := FALSE;
   Sl_DlmKpk_Cls := FALSE;
   Sl_DlmKpk_BthLmt := FALSE;
   Sl_BsltVF_GF := FALSE;
   Sl_BsltVF_Strt := FALSE;
   Sl_BsltVF_Stop := FALSE;
   Sl_BsltVF_Trip := FALSE;
   Sl_BsltKpk_GF := FALSE;
   Sl_BsltKpk_Opn := FALSE;
   Sl_BsltKpk_Cls := FALSE;
   Sl_BsltKpk_BthLmt := FALSE;
   Sl_Ydk := FALSE;
   Sl_Ydk1 := FALSE;
   Hm_DlmHlz_GF := FALSE;
   Hm_DlmHlz_Strt := FALSE;
   Hm_DlmHlz_Stop := FALSE;
   Hm_DlmHlz_Trip := FALSE;
   Hm_Akt_GF := FALSE;
   Hm_Akt_Strt := FALSE;
   Hm_Akt_Stop := FALSE;
   Hm_Akt_Trip := FALSE;
   Hm_SL_HL := FALSE;
   Hm_SL_LL := FALSE;
   Hm_DlmKpk_GF := FALSE;
   Hm_DlmKpk_Opn := FALSE;
   Hm_DlmKpk_Cls := FALSE;
   Hm_DlmKpk_BthLmt := FALSE;
   Hm_BsltVF_GF := FALSE;
   Hm_BsltVF_Strt := FALSE;
   Hm_BsltVF_Stop := FALSE;
   Hm_BsltVF_Trip := FALSE;
   Hm_BsltKpk_GF := FALSE;
   Hm_BsltKpk_Opn := FALSE;
   Hm_BsltKpk_Cls := FALSE;
   Hm_BsltKpk_BthLmt := FALSE;
   Hm_Ydk := FALSE;
   Hm_Ydk1 := FALSE;
   An_DlmHlz_GF := FALSE;
   An_DlmHlz_Strt := FALSE;
   An_DlmHlz_Stop := FALSE;
   An_DlmHlz_Trip := FALSE;
   An_Akt_GF := FALSE;
   An_Akt_Strt := FALSE;
   An_Akt_Stop := FALSE;
   An_Akt_Trip := FALSE;
   An_SL_HL := FALSE;
   An_SL_LL := FALSE;
   An_DlmKpk_GF := FALSE;
   An_DlmKpk_Opn := FALSE;
   An_DlmKpk_Cls := FALSE;
   An_DlmKpk_BthLmt := FALSE;
   An_BsltKrs_GF := FALSE;
   An_BsltKrs_Strt := FALSE;
   An_BsltKrs_Stop := FALSE;
   An_BsltKrs_Trip := FALSE;
   An_BsltHlz_GF := FALSE;
   An_BsltHlz_Strt := FALSE;
   An_BsltHlz_Stop := FALSE;
   An_BsltHlz_Trip := FALSE;
   An_BsltKpk_GF := FALSE;
   An_BsltKpk_Opn := FALSE;
   An_BsltKpk_Cls := FALSE;
   An_BsltKpk_BthLmt := FALSE;
   An_Ydk := FALSE;
   An_Ydk1 := FALSE;
   An_Ydk2 := FALSE;
   An_Ydk3 := FALSE;
   An_Ydk4 := FALSE;
   An_Ydk5 := FALSE;
   e83_TopBnd_GF := FALSE;
   e83_TopBnd_Strt := FALSE;
   e83_TopBnd_Stop := FALSE;
   e83_TopBnd_Trip := FALSE;
   e83_LmtSwtch := FALSE;
   e83_EmrSwtch := FALSE;
   e83_MovingSnsr := FALSE;
   e83_Ydk := FALSE;
   e83_Fan_GF := FALSE;
   e83_Fan_Strt := FALSE;
   e83_Fan_Stop := FALSE;
   e83_Fan_Trip := FALSE;
   e83_Ydk1 := FALSE;
   e83_Ydk2 := FALSE;
   e83_Ydk3 := FALSE;
   e83_Ydk4 := FALSE;
   e87_Bnd_GF := FALSE;
   e87_Bnd_Strt := FALSE;
   e87_Bnd_Stop := FALSE;
   e87_Bnd_Trip := FALSE;
   e87_LmtSwtch := FALSE;
   e87_EmrSwtch := FALSE;
   e87_MovingSnsr := FALSE;
   e87_Ydk := FALSE;
   e87_Fan_GF := FALSE;
   e87_Fan_Strt := FALSE;
   e87_Fan_Stop := FALSE;
   e87_Fan_Trip := FALSE;
   e87_Ydk1 := FALSE;
   e87_Ydk2 := FALSE;
   e87_Ydk3 := FALSE;
   e87_Ydk4 := FALSE;
   TozTopFan_GF1 := FALSE;
   TozTopFan_Strt1 := FALSE;
   TozTopFan_Stop1 := FALSE;
   TozTopFan_Trip1 := FALSE;
   Ydk := FALSE;
   Ydk1 := FALSE;
   Ydk2 := FALSE;
   Ydk3 := FALSE;
   TolErrKmADlm := FALSE;
   TolErrKmABslt := FALSE;
   TolErrKmBDlm := FALSE;
   TolErrKmBBslt := FALSE;
   TolErrSdADlm := FALSE;
   TolErrSdBDlm := FALSE;
   TolErrSdBslt := FALSE;
   TolErrDlADlm := FALSE;
   TolErrDlBDlm := FALSE;
   TolErrDlBslt := FALSE;
   TolErrKlDlm := FALSE;
   TolErrKlBslt := FALSE;
   TolErrFlADlm := FALSE;
   TolErrFlBDlm := FALSE;
   TolErrFlBslt := FALSE;
   TolErrSlDlm := FALSE;
   TolErrSlBslt := FALSE;
   TolErrHmDlm := FALSE;
   TolErrHmBslt := FALSE;
   TolErrAnDlm := FALSE;
   TolErrAnBslt := FALSE;
   TolErrTopKntr := FALSE;
   TolErrYdk := FALSE;
   TolErrYdk1 := FALSE;
   BX3_ErrKmA := FALSE;
   BX3_ErrKmB := FALSE;
   BX3_ErrSd := FALSE;
   BX3_ErrDl := FALSE;
   BX3_ErrKl := FALSE;
   BX3_ErrFl := FALSE;
   BX3_ErrSl := FALSE;
   BX3_ErrHm := FALSE;
   BX3_ErrAn := FALSE;
   BX3_ErrYdk := FALSE;
   BX3_ErrYdk1 := FALSE;
   BX3_ErrYdk2 := FALSE;
   BX3_ErrYdk3 := FALSE;
   BX3_ErrYdk4 := FALSE;
   BX3_ErrYdk5 := FALSE;
   BX3_ErrYdk6 := FALSE;
END_DATA_BLOCK

